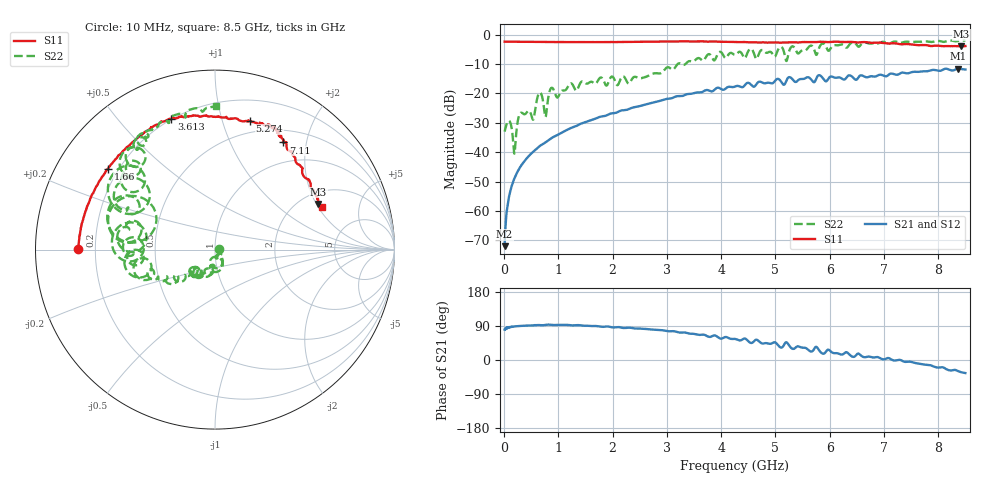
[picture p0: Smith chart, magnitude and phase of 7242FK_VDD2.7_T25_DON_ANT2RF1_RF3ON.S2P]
!Agilent Technologies,E5071C,MY46417908,A.11.23
!Date: Wed Dec 09 15:39:30 2020
!Data & Calibration Information:
!Freq	S11:SOLT2(ON)	S21:SOLT2(ON)	S12:SOLT2(ON)	S22:SOLT2(ON)
!PortZ  Port1:50+j0  Port2:50+j0
!Above PortZ is port z conversion or system Z0 setting when saving the data.
!When reading, reference impedance value at option line is always used.
# Hz S dB R 50
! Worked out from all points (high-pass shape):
!   1601 points, 10 MHz to 8.5 GHz, reference 50 ohm
!   highest |S21| = -11.53 dB at 8.367 GHz (marker M1); lowest = -72.0 dB at 10 MHz (marker M2)
!   |S21| within 3 dB of the highest: 6.31 GHz to 6.427 GHz (117.2 MHz wide, 1.84 % of centre); 6.528 GHz to end of sweep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
!   lowest |S11| = -4.0 dB at 8.426 GHz (marker M3), VSWR 4.41, Z = 123 + j104 ohm
!   |S11| at or under -10 dB: nowhere
!   |S22| runs from -40.5 to -2.0 dB; largest |S21 - S12| = 0.0031
!   S11 on the Smith chart (normalised r, x): 10 MHz: 0.13, +0.00; 1.66 GHz: 0.16, +0.33; 3.613 GHz: 0.20, +0.70; 5.274 GHz: 0.39, +1.23; 7.11 GHz: 0.67, +1.61; 8.5 GHz: 2.67, +2.15
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1e7  -2.35 179.8  -71.96 80.2  -72.93 76.5  -33.00 3.3
8.42875e7  -2.38 178.2  -55.87 86.3  -55.87 86.0  -29.27 -35.2
1.904125e8  -2.39 176.0  -48.91 88.6  -48.89 88.5  -40.50 -45.6
3.230688e8  -2.41 173.1  -44.33 90.1  -44.30 90.3  -26.53 -58.2
5.353188e8  -2.43 168.8  -39.89 91.4  -39.86 91.3  -28.94 -70.8
6.520562e8  -2.45 166.1  -37.98 92.2  -37.99 92.3  -19.73 -80.1
7.634875e8  -2.47 163.8  -36.67 92.5  -36.67 92.6  -28.04 -86.2
8.696125e8  -2.47 161.3  -35.21 92.8  -35.21 92.9  -18.12 -84.0
1.426769e9  -2.52 148.4  -30.19 91.2  -30.19 91.1  -15.96 -107.4
1.660244e9  -2.52 143.0  -28.75 89.7  -28.75 89.7  -16.58 -121.2
2.843538e9  -2.35 119.0  -22.65 79.3  -22.66 79.3  -13.18 -140.0
3.612944e9  -2.28 108.4  -19.63 66.3  -19.63 66.2  -8.17 -162.4
4.255e9  -2.49 97.1  -17.64 55.6  -17.65 55.6  -6.85 -177.2
5.082775e9  -2.72 77.8  -15.45 34.1  -15.42 34.0  -4.22 165.5
5.194206e9  -2.63 75.4  -15.98 46.9  -15.98 46.8  -8.77 153.5
5.2738e9  -2.59 74.8  -14.52 34.2  -14.49 34.3  -4.62 169.8
5.671769e9  -2.55 67.2  -15.57 22.6  -15.52 22.5  -3.78 143.8
7.088538e9  -3.00 57.7  -13.57 5.0  -13.62 4.8  -3.06 124.0
7.109762e9  -3.00 57.5  -13.31 3.6  -13.35 3.7  -2.97 125.4
8.367344e9  -3.90 25.9  -11.53 -29.5  -11.58 -29.5  -2.14 94.4
8.425712e9  -4.01 23.9  -11.67 -32.4  -11.73 -32.5  -2.02 92.4
8.5e9  -3.87 21.8  -11.83 -34.5  -11.91 -34.3  -1.96 89.8
